(* Logix 5000 AddOnInstructionDefinition export AMCI_SD4840E2_Run_Dwell_Move; software revision 20.03 *)

ADD_ON_INSTRUCTION AMCI_SD4840E2_Run_Dwell_Move   (* revision 1.0, vendor AMCI, ExecuteEnableInFalse *)
VAR_INPUT
   Axis_Status_Bits : INT; {required}
   Type_0_for_standard_1_for_indexed : BOOL;
   Assembled_Move_Dwell_Timer : INT; {required}
END_VAR
VAR_IN_OUT
   AMCI_SD4840E2_output_data : _000A:SD4840E2_4342D302:O:0; {required}
END_VAR
VAR_OUTPUT
   EN : BOOL; {visible}
   ER : BOOL; {visible}
END_VAR
VAR
   command_data_block : INT[10];
        [0]   // Command Bits MSW
        [1]   // Command Bits LSW
        [2]   // Upper Target Position
        [3]   // Lower Target Position
        [4]   // Upper Programmed Speed
        [5]   // Lower Programmed Speed
END_VAR

ROUTINE EnableInFalse   (* ladder *)
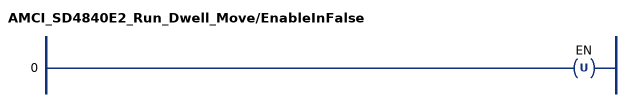
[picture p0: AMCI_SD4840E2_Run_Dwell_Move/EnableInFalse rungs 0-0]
   0: OTU(EN);
END_ROUTINE

ROUTINE Logic   (* ladder *)
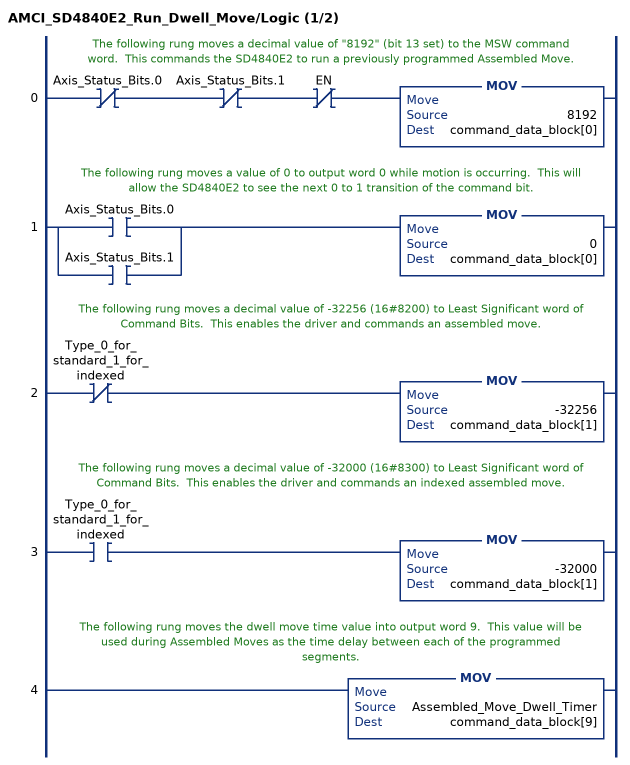
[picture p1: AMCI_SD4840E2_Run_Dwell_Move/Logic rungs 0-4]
   // The following rung moves a decimal value of "8192" (bit 13 set) to the MSW command word.  This commands the SD4840E2 to run a previously programmed Assembled Move.
   0: XIO(Axis_Status_Bits.0)XIO(Axis_Status_Bits.1)XIO(EN)MOV(8192,command_data_block[0]);
   // The following rung moves a value of 0 to output word 0 while motion is occurring.  This will allow the SD4840E2 to see the next 0 to 1 transition of the command bit.
   1: [XIC(Axis_Status_Bits.0) ,XIC(Axis_Status_Bits.1) ]MOV(0,command_data_block[0]);
   // The following rung moves a decimal value of -32256 (16#8200) to Least Significant word of Command Bits.  This enables the driver and commands an assembled move.
   2: XIO(Type_0_for_standard_1_for_indexed)MOV(-32256,command_data_block[1]);
   // The following rung moves a decimal value of -32000 (16#8300) to Least Significant word of Command Bits.  This enables the driver and commands an indexed assembled move.
   3: XIC(Type_0_for_standard_1_for_indexed)MOV(-32000,command_data_block[1]);
   // The following rung moves the dwell move time value into output word 9.  This value will be used during Assembled Moves as the time delay between each of the programmed segments.
   4: MOV(Assembled_Move_Dwell_Timer,command_data_block[9]);
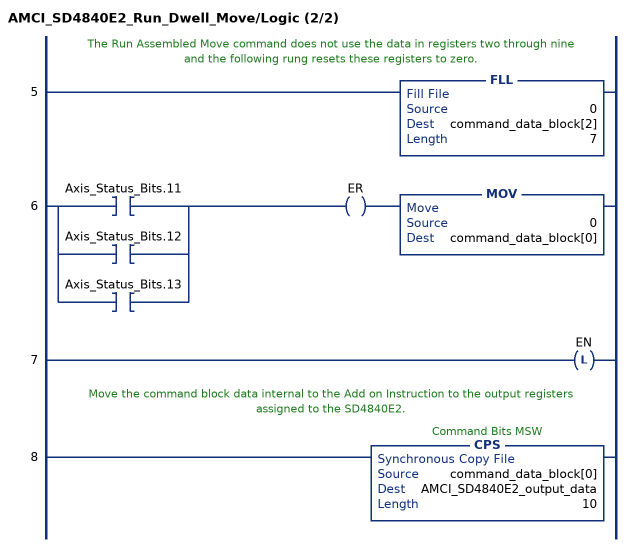
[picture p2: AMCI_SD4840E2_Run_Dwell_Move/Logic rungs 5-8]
   // The Run Assembled Move command does not use the data in registers two through nine and the following rung resets these registers to zero.
   5: FLL(0,command_data_block[2],7);
   6: [XIC(Axis_Status_Bits.11) ,XIC(Axis_Status_Bits.12) ,XIC(Axis_Status_Bits.13) ]OTE(ER)MOV(0,command_data_block[0]);
   7: OTL(EN);
   // Move the command block data internal to the Add on Instruction to the output registers assigned to the SD4840E2.
   8: CPS(command_data_block[0],AMCI_SD4840E2_output_data,10);
END_ROUTINE
END_ADD_ON_INSTRUCTION
